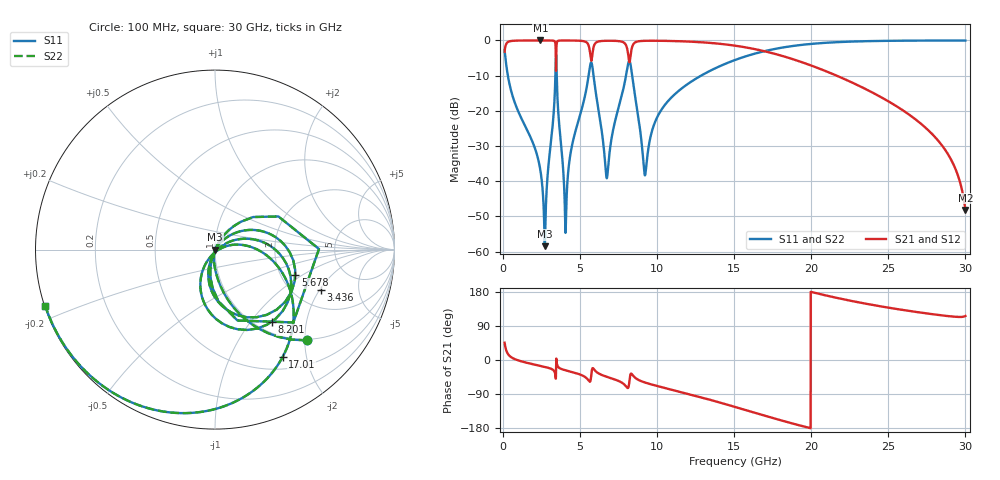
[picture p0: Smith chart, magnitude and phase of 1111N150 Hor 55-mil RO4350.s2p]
# GHz S MA R 50
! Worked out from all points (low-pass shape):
!   3201 points, 100 MHz to 30 GHz, reference 50 ohm
!   highest |S21| = -0.01 dB at 2.417 GHz (marker M1); lowest = -48.2 dB at 30 GHz (marker M2)
!   |S21| within 3 dB of the highest: 104.5 MHz to 3.416 GHz (3.312 GHz wide, 188 % of centre); 8.317 GHz to 16.9 GHz (8.582 GHz wide, 68.1 % of centre)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
!   lowest |S11| = -58.5 dB at 2.707 GHz (marker M3), VSWR 1.00, Z = 50.1 - j0.0457 ohm
!   |S11| at or under -10 dB: 310.8 MHz to 3.396 GHz (3.085 GHz wide, 166 % of centre); 5.871 GHz to 7.977 GHz (2.106 GHz wide, 30.4 % of centre); 8.377 GHz to 12.85 GHz (4.474 GHz wide, 42.2 % of centre)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
!   |S22| runs from -58.5 to 0.0 dB; largest |S21 - S12| = 0
!   S11 on the Smith chart (normalised r, x): 100 MHz: 0.98, -2.06; 3.436 GHz: 2.74, -2.06; 5.678 GHz: 2.39, -0.88; 8.201 GHz: 1.17, -1.28; 17.01 GHz: 0.67, -1.60; 30 GHz: 0.00, -0.16
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0.1  0.7215 -44.5  0.6921 45.5  0.6921 45.5  0.7215 -44.5
0.5298125  0.1895 -82.6  0.9814 7.3  0.9814 7.3  0.1895 -82.6
2.41725  0.01443 -101.6  0.9986 -15.5  0.9986 -15.5  0.01443 -101.6
2.706906  0.001192 -22.5  0.9985 -18.3  0.9985 -18.3  0.001192 -22.5
3.435719  0.632 -21.0  0.3688 -26.8  0.3688 -26.8  0.632 -21.0
4.06175  0.00195 -8.0  0.9977 -27.3  0.9977 -27.3  0.00195 -8.0
4.4355  0.02917 53.8  0.9966 -31.3  0.9966 -31.3  0.02917 53.8
5.089563  0.1029 45.0  0.9847 -39.8  0.9847 -39.8  0.1029 45.0
5.678219  0.4701 -17.8  0.5798 -53.7  0.5798 -53.7  0.4701 -17.8
6.014594  0.183 -100.7  0.9242 -29.8  0.9242 -29.8  0.183 -100.7
6.734063  0.01101 -38.0  0.9883 -44.4  0.9883 -44.4  0.01101 -38.0
7.845969  0.2249 14.5  0.9292 -63.9  0.9292 -63.9  0.2249 14.5
8.201031  0.5116 -52.0  0.4877 -54.6  0.4877 -54.6  0.5116 -52.0
8.472  0.2238 -111.3  0.8949 -42.9  0.8949 -42.9  0.2238 -111.3
9.191469  0.01224 -62.3  0.9868 -59.2  0.9868 -59.2  0.01224 -62.3
10.06978  0.08677 16.2  0.9884 -69.3  0.9884 -69.3  0.08677 16.2
15.05  0.5269 -34.5  0.8421 -123.8  0.8421 -123.8  0.5269 -34.5
17.01219  0.7075 -57.9  0.6975 -147.3  0.6975 -147.3  0.7075 -57.9
20.03956  0.8938 -91.3  0.4363 179.2  0.4363 179.2  0.8938 -91.3
25.01978  0.9868 -132.6  0.1356 138.0  0.1356 138.0  0.9868 -132.6
28.54237  0.9959 -153.9  0.03091 117.4  0.03091 117.4  0.9959 -153.9
30  0.9965 -161.6  0.003888 116.1  0.003888 116.1  0.9965 -161.6
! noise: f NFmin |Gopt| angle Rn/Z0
0.1  0.0008461  0.788  2.413  0.0008211
3.417  0.1305  0.9486  22.95  0.5477
6.743  0.03613  0.6909  44.33  0.01963
10.06  0.03498  0.5709  63.51  0.01096
13.39  0.03805  0.5154  77.79  0.008851
16.7  0.05316  0.5816  91.8  0.01204
20.03  0.08387  0.6972  107.9  0.01987
23.35  0.1558  0.8235  126  0.03958
26.67  0.396  0.9271  144.4  0.1143
30  7.015  0.9948  161.6  11.92
